| IBIS file stm32wba55_ufbga59-smps.ibs
[IBIS ver] 4.2
[File name] stm32wba55_ufbga59-smps.ibs
[File Rev] 1.2
[Date] 22-05-2024
[Source] Data Created at STMicroelectronics
[Notes]  File originated from ELDO simulations.
[Disclaimer]  This information is for modeling purpose only and is
   not guaranteed. The information is subject to change without
   notice.
[Copyright] Copyright 2024 STMicroelectronics Inc.
|   Component stm32wba55_ufbga59-smps
[Component] stm32wba55_ufbga59-smps
[Manufacturer] STMicroelectronics
[Package]
| variable   typ   min   max
R_pkg  0  NA  NA
L_pkg  0  NA  NA
C_pkg  0  NA  NA
[Pin]   signal_name   model_name
A1  VSSSMPS  nc
A2  PB14  io8_ft_100m_v33
A3  PA10  io8_ft_100m_v33
A4  VDDRFPA  nc
A5  OSC_OUT  nc
A6  VDDRF  nc
A7  VSSRF  nc
A8  RF  nc
B1  VDDSMPS  nc
B2  PB13  io8_ft_100m_v33
B3  PA9  io8_ft_100m_v33
B4  VDDHPA  nc
B5  OSC_IN  nc
B6  VDDANA  nc
B7  VSSRF  nc
B8  NRST  ioreset_v33
C1  VLXSMPS  nc
C2  PB12  io8_ft_100m_v33
C3  VDD11  nc
C6  VDD  power
C7  PH3-BOOT0  io8_ft_100m_v33
C8  PB15  io8_ft_100m_v33
D1  PA8  io8_ft_100m_v33
D2  PB11  io8_ft_100m_v33
D4  VSS  gnd
D5  VDD  power
D6  VSS  gnd
D7  PB0  io8_ft_100m_v33
D8  PB1  io8_ft_100m_i2c_v33
E1  PA6  io8_ft_100m_i2c_v33
E2  PA7  io8_ft_100m_i2c_v33
E3  VSS  gnd
E4  VDD  power
E5  VSS  gnd
E7  PB2  io8_ft_100m_i2c_v33
E8  PA11  io8_ft_100m_v33
F1  VDDA  nc
F2  VSSA  nc
F3  PA5  io8_ft_100m_v33
F5  VDD  power
F6  PA14  io8_ft_100m_v33
F7  PA12  io8_ft_100m_v33
F8  PA13  io8_ft_100m_v33
G1  PA4  io8_ft_100m_v33
G2  PA3  io8_ft_100m_v33
G3  PA2  io8_ft_100m_v33
G4  PC15-OSC32_OUT  io8_ft_100m_tamp
G5  PC13  io8_ft_100m_v33
G6  PB6  io8_ft_100m_v33
G7  PB3  io8_ft_100m_i2c_v33
G8  PA15  io8_ft_100m_i2c_v33
H1  PA0  io8_ft_100m_v33
H2  PA1  io8_ft_100m_v33
H3  PB9  io8_ft_100m_v33
H4  PC14-OSC32_IN  io8_ft_100m_tamp
H5  PB8  io8_ft_100m_v33
H6  PB7  io8_ft_100m_v33
H7  PB5  io8_ft_100m_v33
H8  PB4  io8_ft_100m_v33
[Package Model]   492-bga-5x5-59-100mhz-240318
[Pin Mapping]   pulldown_ref   pullup_ref   | Comment
A1  nc  nc
A2  gndio  vddiom
A3  gndio  vddiom
A4  nc  nc
A5  nc  nc
A6  nc  nc
A7  nc  nc
A8  nc  nc
B1  nc  nc
B2  gndio  vddiom
B3  gndio  vddiom
B4  nc  nc
B5  nc  nc
B6  nc  nc
B7  nc  nc
B8  gndio  vddiom
C1  nc  nc
C2  gndio  vddiom
C3  nc  nc
C6  nc  vddiom
C7  gndio  vddiom
C8  gndio  vddiom
D1  gndio  vddiom
D2  gndio  vddiom
D4  gndio  nc
D5  nc  vddiom
D6  gndio  nc
D7  gndio  vddiom
D8  gndio  vddiom
E1  gndio  vddiom
E2  gndio  vddiom
E3  gndio  nc
E4  nc  vddiom
E5  gndio  nc
E7  gndio  vddiom
E8  gndio  vddiom
F1  nc  nc
F2  nc  nc
F3  gndio  vddiom
F5  nc  vddiom
F6  gndio  vddiom
F7  gndio  vddiom
F8  gndio  vddiom
G1  gndio  vddiom
G2  gndio  vddiom
G3  gndio  vddiom
G4  gndio  vddiom
G5  gndio  vddiom
G6  gndio  vddiom
G7  gndio  vddiom
G8  gndio  vddiom
H1  gndio  vddiom
H2  gndio  vddiom
H3  gndio  vddiom
H4  gndio  vddiom
H5  gndio  vddiom
H6  gndio  vddiom
H7  gndio  vddiom
H8  gndio  vddiom
[Model Selector] io8_ft_100m_i2c_v33
io8_ft_100m_v33_ls_1v2  "GPIO_V33 100MHz - 5V tolerant - low speed - 1.2V range"
io8_ft_100m_v33_ls_1v8  "GPIO_V33 100MHz - 5V tolerant - low speed - 1.8V range"
io8_ft_100m_v33_ls_3v3  "GPIO_V33 100MHz - 5V tolerant - low speed - 3.3V range"
io8_ft_100m_v33_ms_1v2  "GPIO_V33 100MHz - 5V tolerant - med speed - 1.2V range"
io8_ft_100m_v33_ms_1v8  "GPIO_V33 100MHz - 5V tolerant - med speed - 1.8V range"
io8_ft_100m_v33_ms_3v3  "GPIO_V33 100MHz - 5V tolerant - med speed - 3.3V range"
io8_ft_100m_v33_fs_1v2  "GPIO_V33 100MHz - 5V tolerant - fast speed - 1.2V range"
io8_ft_100m_v33_fs_1v8  "GPIO_V33 100MHz - 5V tolerant - fast speed - 1.8V range"
io8_ft_100m_v33_fs_3v3  "GPIO_V33 100MHz - 5V tolerant - fast speed - 3.3V range"
io8_ft_100m_v33_hs_1v2  "GPIO_V33 100MHz - 5V tolerant - high speed - 1.2V range"
io8_ft_100m_v33_hs_1v8  "GPIO_V33 100MHz - 5V tolerant - high speed - 1.8V range"
io8_ft_100m_v33_hs_3v3  "GPIO_V33 100MHz - 5V tolerant - high speed - 3.3V range"
io8_ft_100m_i2c_v33_ls_1v2  "GPIO_V33 100MHz with I2C open-drain - 5V tolerant - low speed - 1.2V range"
io8_ft_100m_i2c_v33_ls_1v8  "GPIO_V33 100MHz with I2C open-drain - 5V tolerant - low speed - 1.8V range"
io8_ft_100m_i2c_v33_ls_3v3  "GPIO_V33 100MHz with I2C open-drain - 5V tolerant - low speed - 3.3V range"
io8_ft_100m_i2c_v33_ms_1v2  "GPIO_V33 100MHz with I2C open-drain - 5V tolerant - med speed - 1.2V range"
io8_ft_100m_i2c_v33_ms_1v8  "GPIO_V33 100MHz with I2C open-drain - 5V tolerant - med speed - 1.8V range"
io8_ft_100m_i2c_v33_ms_3v3  "GPIO_V33 100MHz with I2C open-drain - 5V tolerant - med speed - 3.3V range"
io8_ft_100m_i2c_v33_fs_1v2  "GPIO_V33 100MHz with I2C open-drain - 5V tolerant - fast speed - 1.2V range"
io8_ft_100m_i2c_v33_fs_1v8  "GPIO_V33 100MHz with I2C open-drain - 5V tolerant - fast speed - 1.8V range"
io8_ft_100m_i2c_v33_fs_3v3  "GPIO_V33 100MHz with I2C open-drain - 5V tolerant - fast speed - 3.3V range"
io8_ft_100m_i2c_v33_hs_1v2  "GPIO_V33 100MHz with I2C open-drain - 5V tolerant - high speed - 1.2V range"
io8_ft_100m_i2c_v33_hs_1v8  "GPIO_V33 100MHz with I2C open-drain - 5V tolerant - high speed - 1.8V range"
io8_ft_100m_i2c_v33_hs_3v3  "GPIO_V33 100MHz with I2C open-drain - 5V tolerant - high speed - 3.3V range"
io8_ft_100m_i2c_fmp_v33_3v3  "GPIO_V33 100MHz with I2C fm+ open-drain - 5V tolerant - low speed - 3.3V range"
[Model Selector] io8_ft_100m_tamp
io8_ft_100m_ls_1v2 "GPIO SPI - 5V tolerant - low speed - 1.2V range"
io8_ft_100m_ls_1v8 "GPIO SPI - 5V tolerant - low speed - 1.8V range"
io8_ft_100m_ls_3v3 "GPIO SPI - 5V tolerant - low speed - 3.3V range"
io8_ft_100m_ms_1v2 "GPIO SPI - 5V tolerant - med speed - 1.2V range"
io8_ft_100m_ms_1v8 "GPIO SPI - 5V tolerant - med speed - 1.8V range"
io8_ft_100m_ms_3v3 "GPIO SPI - 5V tolerant - med speed - 3.3V range"
io8_ft_100m_fs_1v2 "GPIO SPI - 5V tolerant - fast speed - 1.2V range"
io8_ft_100m_fs_1v8 "GPIO SPI - 5V tolerant - fast speed - 1.8V range"
io8_ft_100m_fs_3v3 "GPIO SPI - 5V tolerant - fast speed - 3.3V range"
io8_ft_100m_hs_1v2 "GPIO SPI - 5V tolerant - high speed - 1.2V range"
io8_ft_100m_hs_1v8 "GPIO SPI - 5V tolerant - high speed - 1.8V range"
io8_ft_100m_hs_3v3 "GPIO SPI - 5V tolerant - high speed - 3.3V range"
io8_ft_tamp_ls_1v2 "IO TAMPER_3V - 5V tolerant - low speed - 1.2V range"
io8_ft_tamp_ls_1v8 "IO TAMPER_3V - 5V tolerant - low speed - 1.8V range"
io8_ft_tamp_ls_3v3 "IO TAMPER_3V-  5V tolerant - low speed - 3.3V range"
io8_ft_tamp_ms_1v2 "IO TAMPER_3V - 5V tolerant - med speed - 1.2V range"
io8_ft_tamp_ms_1v8 "IO TAMPER_3V - 5V tolerant - med speed - 1.8V range"
io8_ft_tamp_ms_3v3 "IO TAMPER_3V - 5V tolerant - med speed - 3.3V range"
io8_ft_tamp_fs_1v2 "IO TAMPER_3V - 5V tolerant - fast speed - 1.2V range"
io8_ft_tamp_fs_1v8 "IO TAMPER_3V - 5V tolerant - fast speed - 1.8V range"
io8_ft_tamp_fs_3v3 "IO TAMPER_3V - 5V tolerant - fast speed - 3.3V range"
io8_ft_tamp_hs_1v2 "IO TAMPER_3V - 5V tolerant - high speed - 1.2V range"
io8_ft_tamp_hs_1v8 "IO TAMPER_3V - 5V tolerant - high speed - 1.8V range"
io8_ft_tamp_hs_3v3 "IO TAMPER_3V - 5V tolerant - high speed - 3.3V range"
[Model Selector] io8_ft_100m_v33
io8_ft_100m_v33_ls_1v2  "GPIO_V33 100MHz - 5V tolerant - low speed - 1.2V range"
io8_ft_100m_v33_ls_1v8  "GPIO_V33 100MHz - 5V tolerant - low speed - 1.8V range"
io8_ft_100m_v33_ls_3v3  "GPIO_V33 100MHz - 5V tolerant - low speed - 3.3V range"
io8_ft_100m_v33_ms_1v2  "GPIO_V33 100MHz - 5V tolerant - med speed - 1.2V range"
io8_ft_100m_v33_ms_1v8  "GPIO_V33 100MHz - 5V tolerant - med speed - 1.8V range"
io8_ft_100m_v33_ms_3v3  "GPIO_V33 100MHz - 5V tolerant - med speed - 3.3V range"
io8_ft_100m_v33_fs_1v2  "GPIO_V33 100MHz - 5V tolerant - fast speed - 1.2V range"
io8_ft_100m_v33_fs_1v8  "GPIO_V33 100MHz - 5V tolerant - fast speed - 1.8V range"
io8_ft_100m_v33_fs_3v3  "GPIO_V33 100MHz - 5V tolerant - fast speed - 3.3V range"
io8_ft_100m_v33_hs_1v2  "GPIO_V33 100MHz - 5V tolerant - high speed - 1.2V range"
io8_ft_100m_v33_hs_1v8  "GPIO_V33 100MHz - 5V tolerant - high speed - 1.8V range"
io8_ft_100m_v33_hs_3v3  "GPIO_V33 100MHz - 5V tolerant - high speed - 3.3V range"
[Model Selector] ioreset_v33
ioreset_v33_1v2 "Reset PAD. 5V tolerant. 1.2V range"
ioreset_v33_1v8 "Reset PAD. 5V tolerant. 1.8V range"
ioreset_v33_3v3 "Reset PAD. 5V tolerant. 3.3V range"
[Define Package Model]  492-bga-5x5-59-100mhz-240318
[Manufacturer]  unknown
[OEM]  unknown
[Description]  unknown
[Number Of Pins]  52
[Pin Numbers]
| Pin Name Terminal   Net Name   Starting Node   Ending Node
A8 | ANT_RF
B8 | NRST
B5 | OSC_IN
A5 | OSC_OUT
H1 | PA0
H2 | PA1
G3 | PA2
G2 | PA3
G1 | PA4
F3 | PA5
E1 | PA6
E2 | PA7
D1 | PA8
B3 | PA9
A3 | PA10
E8 | PA11
F7 | PA12
F8 | PA13
F6 | PA14
G8 | PA15
D7 | PB0
D8 | PB1
E7 | PB2
G7 | PB3
H8 | PB4
H7 | PB5
G6 | PB6
H6 | PB7
H5 | PB8
H3 | PB9
D2 | PB11
C2 | PB12
B2 | PB13
A2 | PB14
C8 | PB15
G5 | PC13
H4 | PC14-OSC32_IN
G4 | PC15-OSC32_OUT
C7 | PH3-BOOT0
C3 | VDD11
A6 | VDDRF
C6 | VDD
F1 | VDDA
B6 | VDDANA
B4 | VDDHPA
A4 | VDDRFPA
B1 | VDDSMPS
C1 | VLXSMPS
D4 | VSS
F2 | VSSA
A1 | VSSSMPS
A7 | VSSRF
|[Merged Pins]  C6
|D5  |  VDD
|E4  |  VDD
|F5  |  VDD
|[Merged Pins]  D4
|D6  |  VSS
|E3  |  VSS
|E5  |  VSS
|[Merged Pins]  A7
|B7  |  VSSRF
[Model Data]
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[End Model Data]
[End Package Model]
|End [Component]
| Models and submodels in the file (52): io8_ft_100m_fs_1v2 (I/O), io8_ft_100m_fs_1v8 (I/O), io8_ft_100m_fs_3v3 (I/O), io8_ft_100m_hs_1v2 (I/O), io8_ft_100m_hs_1v8 (I/O), io8_ft_100m_hs_3v3 (I/O), io8_ft_100m_i2c_fmp_v33_3v3 (I/O_open_drain), io8_ft_100m_i2c_v33_fs_1v2 (I/O_open_drain), io8_ft_100m_i2c_v33_fs_1v8 (I/O_open_drain), io8_ft_100m_i2c_v33_fs_3v3 (I/O_open_drain), io8_ft_100m_i2c_v33_hs_1v2 (I/O_open_drain), io8_ft_100m_i2c_v33_hs_1v8 (I/O_open_drain), io8_ft_100m_i2c_v33_hs_3v3 (I/O_open_drain), io8_ft_100m_i2c_v33_ls_1v2 (I/O_open_drain), io8_ft_100m_i2c_v33_ls_1v8 (I/O_open_drain), io8_ft_100m_i2c_v33_ls_3v3 (I/O_open_drain), io8_ft_100m_i2c_v33_ms_1v2 (I/O_open_drain), io8_ft_100m_i2c_v33_ms_1v8 (I/O_open_drain), io8_ft_100m_i2c_v33_ms_3v3 (I/O_open_drain), io8_ft_100m_ls_1v2 (I/O), io8_ft_100m_ls_1v8 (I/O), io8_ft_100m_ls_3v3 (I/O), io8_ft_100m_ms_1v2 (I/O), io8_ft_100m_ms_1v8 (I/O), io8_ft_100m_ms_3v3 (I/O), io8_ft_100m_v33_fs_1v2 (I/O), io8_ft_100m_v33_fs_1v8 (I/O), io8_ft_100m_v33_fs_3v3 (I/O), io8_ft_100m_v33_hs_1v2 (I/O), io8_ft_100m_v33_hs_1v8 (I/O), io8_ft_100m_v33_hs_3v3 (I/O), io8_ft_100m_v33_ls_1v2 (I/O), io8_ft_100m_v33_ls_1v8 (I/O), io8_ft_100m_v33_ls_3v3 (I/O), io8_ft_100m_v33_ms_1v2 (I/O), io8_ft_100m_v33_ms_1v8 (I/O), io8_ft_100m_v33_ms_3v3 (I/O), io8_ft_tamp_fs_1v2 (I/O), io8_ft_tamp_fs_1v8 (I/O), io8_ft_tamp_fs_3v3 (I/O), io8_ft_tamp_hs_1v2 (I/O), io8_ft_tamp_hs_1v8 (I/O), io8_ft_tamp_hs_3v3 (I/O), io8_ft_tamp_ls_1v2 (I/O), io8_ft_tamp_ls_1v8 (I/O), io8_ft_tamp_ls_3v3 (I/O), io8_ft_tamp_ms_1v2 (I/O), io8_ft_tamp_ms_1v8 (I/O), io8_ft_tamp_ms_3v3 (I/O), ioreset_v33_1v2 (I/O_open_drain), ioreset_v33_1v8 (I/O_open_drain), ioreset_v33_3v3 (I/O_open_drain)
